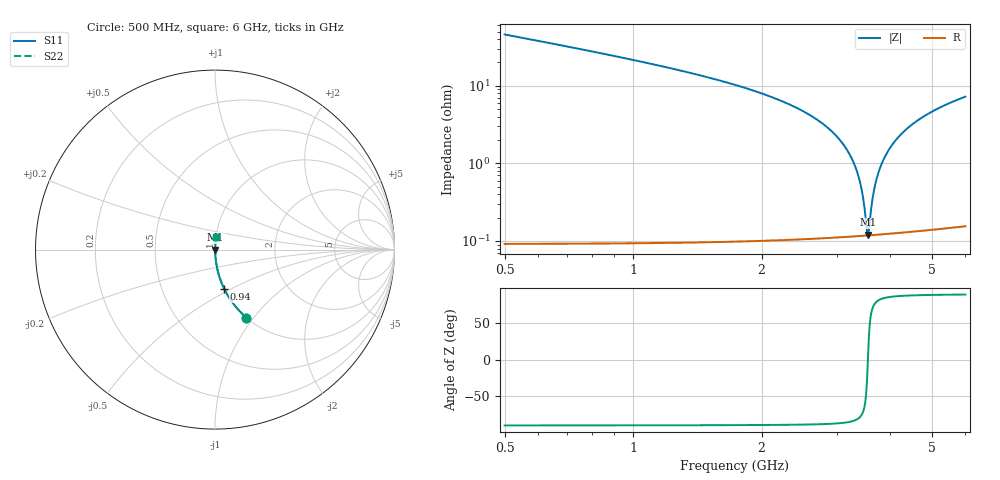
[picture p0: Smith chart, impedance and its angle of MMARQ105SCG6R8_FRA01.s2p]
! MMARQ105SCG6R8_FRA01  S-PARAMETER MODEL  ( General Type )
! Model Generated by TAIYO YUDEN Corporation (http://www.ty-top.com)
! Version 1.0
! TAIYO YUDEN Control No. 200326
! Copyright(c) 2020 TAIYO YUDEN CO.,LTD. All Rights Reserved.
! Product Description (link to TY-COMPAS)
! https://ds.yuden.co.jp/TYCOMPAS/or/detail?pn=MMARQ105SCG6R8CFRA01&u=M
! Products Name : Multilayer Ceramic Capacitors
! Characteristics :
!  Capacitance : 6.8 pF , Rated Voltage : 250V , TCC : CG / C0G
!  Case Size : 1.0 x 0.5 / 0.039 x 0.02 [mm/inch] , Thickness : 0.5 / 0.02 [mm/inch]
!  (Conditions: Temperature = 25 degC , DC Bias Current/Voltage = 0A / 0V)
! External Node Assignments :
!  1  o---| |---o  2
! GND o---------o GND
! Frequency Range : 500MHz  -  6GHz  [ 401 STEP ]
# MHz S RI R 50
! Freq[MHz].  S11 Real  S11 Imag  S21 Real  S21 Imag  S12 Real  S12 Imag  S22 Real  S22 Imag
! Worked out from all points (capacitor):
!   401 points, 500 MHz to 6 GHz, reference 50 ohm
!   read as one part in series: C = 6.79 pF near 527.5 MHz
!   lowest |Z| = 120 mohm at 3.553 GHz (marker M1)
!   series resonance near 3.547 GHz, so ESL is about 300 pH
!   S11 on the Smith chart (normalised r, x): 500 MHz: 1.00, -0.92; 940 MHz: 1.00, -0.46; 6 GHz: 1.00, +0.15
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500  0.1748 -0.3788  0.8252 0.3788  0.8252 0.3788  0.1748 -0.3788
692.5  0.0965 -0.2938  0.9035 0.2938  0.9035 0.2938  0.0965 -0.2938
940  0.0518 -0.2196  0.9482 0.2196  0.9482 0.2196  0.0518 -0.2196
1421.25  0.0197 -0.1355  0.9803 0.1355  0.9803 0.1355  0.0197 -0.1355
2342.5  0.00419 -0.0561  0.9958 0.0561  0.9958 0.0561  0.00419 -0.0561
2906.25  0.00179 -0.0264  0.9982 0.0264  0.9982 0.0264  0.00179 -0.0264
3098.75  0.00144 -0.0178  0.9986 0.0178  0.9986 0.0178  0.00144 -0.0178
3250  0.00127 -0.0115  0.9987 0.0115  0.9987 0.0115  0.00127 -0.0115
3332.5  0.00122 -0.0082  0.9988 0.0082  0.9988 0.0082  0.00122 -0.0082
3401.25  0.00119 -0.00551  0.9988 0.00551  0.9988 0.00551  0.00119 -0.00551
3456.25  0.00118 -0.0034  0.9988 0.0034  0.9988 0.0034  0.00118 -0.0034
3525  0.00118 -0.000801  0.9988 0.000801  0.9988 0.000801  0.00118 -0.000801
3552.5  0.00118 0.000222  0.9988 -0.000222  0.9988 -0.000222  0.00118 0.000222
3566.25  0.00118 0.000731  0.9988 -0.000731  0.9988 -0.000731  0.00118 0.000731
3621.25  0.0012 0.00275  0.9988 -0.00275  0.9988 -0.00275  0.0012 0.00275
3662.5  0.00121 0.00424  0.9988 -0.00424  0.9988 -0.00424  0.00121 0.00424
3758.75  0.00127 0.00766  0.9987 -0.00766  0.9987 -0.00766  0.00127 0.00766
3923.75  0.00141 0.0133  0.9986 -0.0133  0.9986 -0.0133  0.00141 0.0133
4171.25  0.00173 0.0214  0.9983 -0.0214  0.9983 -0.0214  0.00173 0.0214
4556.25  0.00243 0.0333  0.9976 -0.0333  0.9976 -0.0333  0.00243 0.0333
5092.5  0.00377 0.0485  0.9962 -0.0485  0.9962 -0.0485  0.00377 0.0485
6000  0.00675 0.0719  0.9932 -0.0719  0.9932 -0.0719  0.00675 0.0719
